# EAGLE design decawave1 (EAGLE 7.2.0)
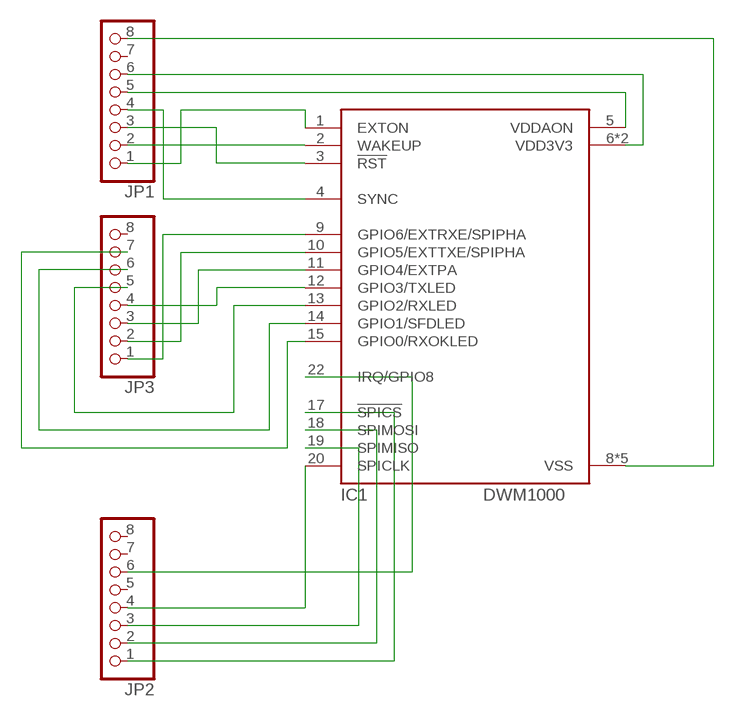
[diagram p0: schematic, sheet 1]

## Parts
IC1  DWM1000  [DWM1000]
JP1  PINHD-1X8_2.00  [1X08M]
JP2  PINHD-1X8_2.00  [1X08M]
JP3  PINHD-1X8_2.00  [1X08M]

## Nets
N$1: IC1.3(!RST) JP1.3
N$2: IC1.2(WAKEUP) JP1.2
N$3: IC1.1(EXTON) JP1.1
N$4: IC1.4(SYNC) JP1.4
N$5: IC1.5(VDDAON) JP1.5
N$6: IC1.6(VDD3V3) IC1.7(VDD3V3) JP1.6
N$7: IC1.8(VSS) IC1.16(VSS) IC1.21(VSS) IC1.23(VSS) IC1.24(VSS) JP1.8
N$8: IC1.9(GPIO6/EXTRXE/SPIPHA) JP3.1
N$9: IC1.10(GPIO5/EXTTXE/SPIPHA) JP3.2
N$10: IC1.11(GPIO4/EXTPA) JP3.3
N$11: IC1.12(GPIO3/TXLED) JP3.4
N$12: IC1.13(GPIO2/RXLED) JP3.5
N$13: IC1.14(GPIO1/SFDLED) JP3.6
N$14: IC1.15(GPIO0/RXOKLED) JP3.7
N$15: IC1.20(SPICLK) JP2.4
N$16: IC1.19(SPIMISO) JP2.3
N$17: IC1.18(SPIMOSI) JP2.2
N$18: IC1.17(!SPICS) JP2.1
N$19: IC1.22(IRQ/GPIO8) JP2.6
Unconnected: JP1.7 JP2.5 JP2.7 JP2.8 JP3.8

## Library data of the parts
IC1 = decawave:DWM1000
JP1-JP3 = con-pinhead:PINHD-1X8: PIN HEADER

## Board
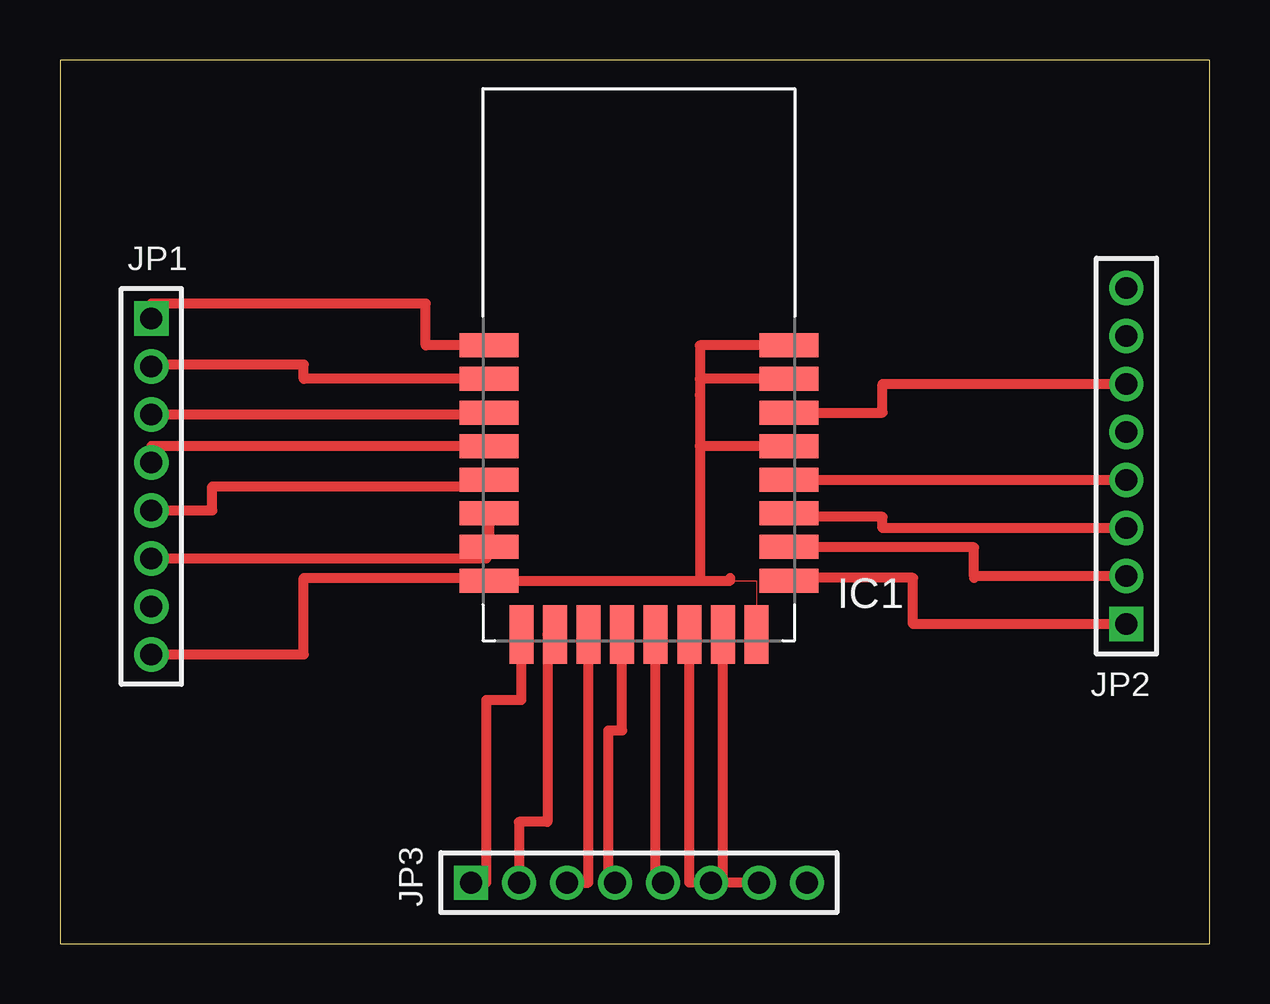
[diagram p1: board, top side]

Size 47.93 x 36.82 mm. Coordinates in mm from the lower left corner, seen from the top.
Outline: 0,0 47.93,0 47.93,36.82 0,36.82 0,0
Copper layers (1*16): Top 0.035mm / dielectric 1.5mm / Bottom 0.035mm
Design rules "default": minimum track width 10mil, minimum drill 24mil, track to track 8mil, track to pad 8mil, pad to pad 8mil, via to via 8mil, smd to smd 8mil, copper to edge 40mil, drill to drill 8mil, minimum pad ring 10mil, minimum via ring 8mil, stop-mask expansion 4mil, vias tented up to drill 0mil, thermal gap 10mil

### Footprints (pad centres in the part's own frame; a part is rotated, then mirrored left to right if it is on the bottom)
DWM1000 = smd 2.45 x 1: 1 -6.25,0.8; 2 -6.25,-0.6; 3 -6.25,-2; 4 -6.25,-3.4; 5 -6.25,-4.8; 6 -6.25,-6.2; 7 -6.25,-7.6; 8 -6.25,-9; 17 6.25,-9; 18 6.25,-7.6; 19 6.25,-6.2; 20 6.25,-4.8; 21 6.25,-3.4; 22 6.25,-2; 23 6.25,-0.6; 24 6.25,0.8 | smd 1 x 2.45: 9 -4.9,-11.25; 10 -3.5,-11.25; 11 -2.1,-11.25; 12 -0.7,-11.25; 13 0.7,-11.25; 14 2.1,-11.25; 15 3.5,-11.25; 16 4.9,-11.25
1X08M = drill 0.914 square: 1 -7,0 | drill 0.914: 2 -5,0; 3 -3,0; 4 -1,0; 5 1,0; 6 3,0; 7 5,0; 8 7,0

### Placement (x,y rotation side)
IC1  24.13,24.13 0 top
JP1  3.81,19.05 270 top
JP2  44.45,20.32 90 top
JP3  24.13,2.54 0 top

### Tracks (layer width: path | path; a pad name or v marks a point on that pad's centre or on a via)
GND
  pour Top (isolate 20.32): 48.26,36.83 0,36.83 0,0 48.26,0
N$1
  Top 0.406: JP1.3 17.88,22.05 IC1.3
N$2
  Top 0.406: IC1.2 10.16,23.53 10.16,24.13 3.81,24.13 JP1.2
N$3
  Top 0.406: IC1.1 15.24,24.93 15.24,26.67 3.81,26.67 JP1.1
N$4
  Top 0.406: IC1.4 3.81,20.73 JP1.4
N$5
  Top 0.406: JP1.5 6.35,18.05 6.35,19.05 17.88,19.05 IC1.5
N$6
  Top 0.406: JP1.6 17.78,16.05 17.78,16.51 17.88,16.51 IC1.7 IC1.6
N$7
  Top 0: 27.94,15.13 29.03,15.13 IC1.16
  Top 0.406: JP1.8 10.16,12.05 10.16,15.24 17.88,15.24 IC1.8 26.67,15.13 | 26.67,15.13 27.94,15.13 27.94,15.24 | IC1.21 26.67,20.73 | 26.67,20.73 26.67,15.13 | IC1.24 26.67,24.93 26.67,23.53 | 26.67,20.73 26.67,22.86 26.67,23.53 | IC1.23 26.67,23.53
N$8
  Top 0.406: JP3.1 17.78,2.54 17.78,10.16 19.23,10.16 IC1.9
N$9
  Top 0.406: IC1.10 20.32,12.88 20.32,5.08 19.13,5.08 JP3.2
N$10
  Top 0.406: JP3.3 22.03,2.54 IC1.11
N$11
  Top 0.406: JP3.4 22.86,2.54 22.86,8.89 23.43,8.89 IC1.12
N$12
  Top 0.406: JP3.5 24.83,2.54 IC1.13
N$13
  Top 0.406: JP3.6 26.23,2.54 IC1.14
N$14
  Top 0.406: JP3.7 27.63,2.54 IC1.15
N$15
  Top 0.406: JP2.4 IC1.20
N$16
  Top 0.406: JP2.3 34.29,17.32 34.29,17.78 30.38,17.78 IC1.19
N$17
  Top 0.406: JP2.2 38.1,15.32 | 38.1,15.32 38.1,15.24 | 38.1,15.32 38.1,16.51 30.38,16.51 IC1.18
N$18
  Top 0.406: JP2.1 35.56,13.32 35.56,15.24 30.38,15.24 IC1.17
N$19
  Top 0.406: JP2.6 34.29,23.32 34.29,22.13 IC1.22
